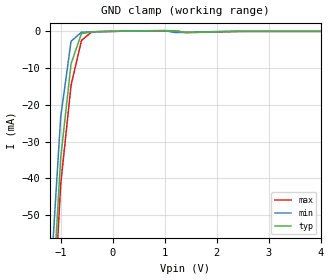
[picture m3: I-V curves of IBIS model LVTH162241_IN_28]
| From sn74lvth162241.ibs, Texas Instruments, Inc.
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|   Model LVTH162241 Input_IN_28
[Model]   LVTH162241_IN_28
Model_type  Input
Polarity   Non-Inverting
Vinl = 0.8V
Vinh = 2.0V
| variable   typ   min   max
C_comp   4pf   NA   NA
[Temperature Range]   40   -25   100
| Ambient temperature   25   -40   85
[Voltage range]   2.8   2.7   2.9
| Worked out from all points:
|   GND clamp passes 1 mA (typ) near -0.61 V on its own axis
[GND Clamp]
|   Voltage   I(typ)   I(min)   I(max)
-5V       -1.699A    -1.78A     -1.549A
-1.2V     -83.48mA   -69.18mA   -94.33mA
-1V       -34.51mA   -23.32mA   -41.69mA
-800mV    -8.788mA   -2.684mA   -14.67mA
-600mV    -612.4uA   -219.4uA   -2.449mA
-400mV    -105.1uA   -123.1uA   -132uA
-200mV    -50.77uA   -60.21uA   -44.53uA
1V        188.1uA    223.5uA    166.5uA
1.2V      172.1uA    -326.2uA   164.9uA
1.4V      -307.4uA   -280.4uA   -320.2uA
2.4V      -640.6nA   -1.291nA   -29.26uA
5V        196.6pA    1.139nA    -78.08pA
